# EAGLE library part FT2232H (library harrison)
FT2232H USB to FIFO
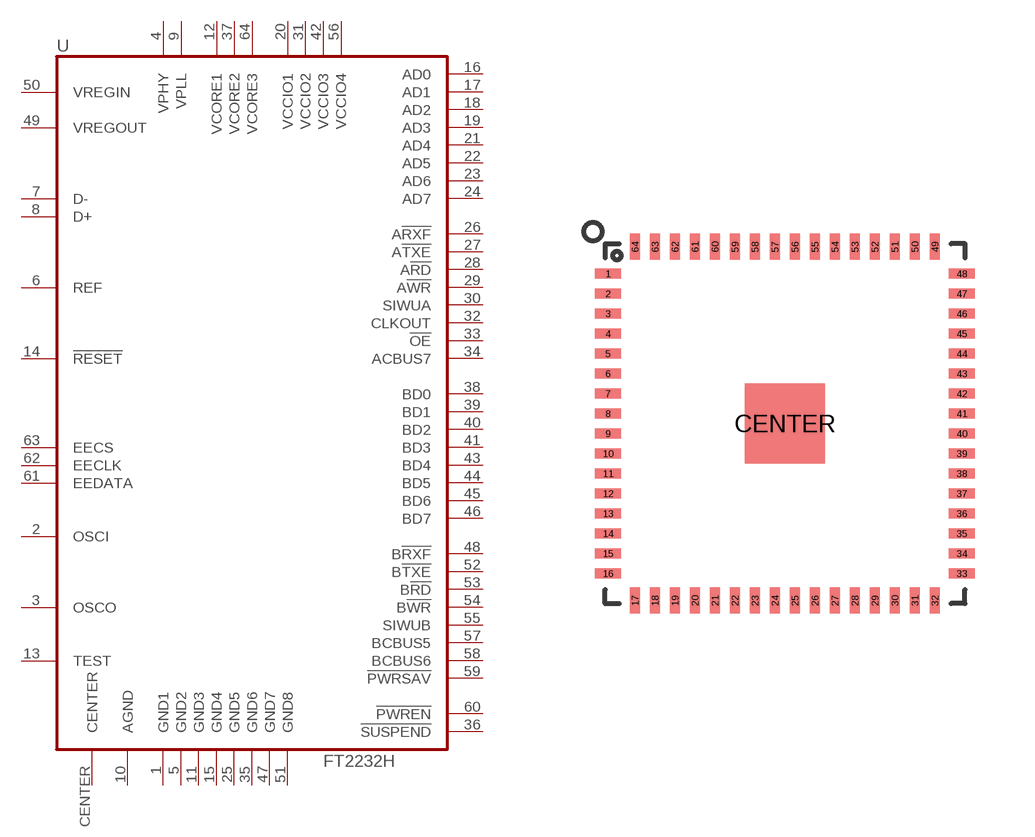
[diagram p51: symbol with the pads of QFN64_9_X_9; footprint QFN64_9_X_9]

Designator prefix U

## FT2232H  [QFN64_9_X_9]
1  GND1  pwr
2  OSCI  in
3  OSCO  out
4  VPHY  pwr
5  GND2  pwr
6  REF  pas
7  D-
8  D+
9  VPLL  pwr
10  AGND  pwr
11  GND3  pwr
12  VCORE1  pwr
13  TEST  in
14  !RESET!  in
15  GND4  pwr
16  AD0
17  AD1
18  AD2
19  AD3
20  VCCIO1  pwr
21  AD4
22  AD5
23  AD6
24  AD7
25  GND5  pwr
26  A!RXF!  out
27  A!TXE!  out
28  A!RD!  in
29  A!WR!  in
30  SIWUA  in
31  VCCIO2  pwr
32  CLKOUT  out
33  !OE!  in
34  ACBUS7
35  GND6  pwr
36  !SUSPEND!  out
37  VCORE2  pwr
38  BD0
39  BD1
40  BD2
41  BD3
42  VCCIO3  pwr
43  BD4
44  BD5
45  BD6
46  BD7
47  GND7  pwr
48  B!RXF!  out
49  VREGOUT  pwr
50  VREGIN  pwr
51  GND8  pwr
52  B!TXE!  out
53  B!RD!  in
54  B!WR!  in
55  SIWUB  in
56  VCCIO4  pwr
57  BCBUS5
58  BCBUS6
59  !PWRSAV!  in
60  !PWREN!  out
61  EEDATA
62  EECLK  out
63  EECS
64  VCORE3  pwr
CENTER  CENTER  pwr

## Footprint QFN64_9_X_9 (pad centres in mm)
smd 0.65 x 0.25: 1 -4.425,3.75; 2 -4.425,3.25; 3 -4.425,2.75; 4 -4.425,2.25; 5 -4.425,1.75; 6 -4.425,1.25; 7 -4.425,0.75; 8 -4.425,0.25; 9 -4.425,-0.25; 10 -4.425,-0.75; 11 -4.425,-1.25; 12 -4.425,-1.75; 13 -4.425,-2.25; 14 -4.425,-2.75; 15 -4.425,-3.25; 16 -4.425,-3.75; 33 4.425,-3.75; 34 4.425,-3.25; 35 4.425,-2.75; 36 4.425,-2.25; 37 4.425,-1.75; 38 4.425,-1.25; 39 4.425,-0.75; 40 4.425,-0.25; 41 4.425,0.25; 42 4.425,0.75; 43 4.425,1.25; 44 4.425,1.75; 45 4.425,2.25; 46 4.425,2.75; 47 4.425,3.25; 48 4.425,3.75
smd 0.25 x 0.65: 17 -3.75,-4.425; 18 -3.25,-4.425; 19 -2.75,-4.425; 20 -2.25,-4.425; 21 -1.75,-4.425; 22 -1.25,-4.425; 23 -0.75,-4.425; 24 -0.25,-4.425; 25 0.25,-4.425; 26 0.75,-4.425; 27 1.25,-4.425; 28 1.75,-4.425; 29 2.25,-4.425; 30 2.75,-4.425; 31 3.25,-4.425; 32 3.75,-4.425; 49 3.75,4.425; 50 3.25,4.425; 51 2.75,4.425; 52 2.25,4.425; 53 1.75,4.425; 54 1.25,4.425; 55 0.75,4.425; 56 0.25,4.425; 57 -0.25,4.425; 58 -0.75,4.425; 59 -1.25,4.425; 60 -1.75,4.425; 61 -2.25,4.425; 62 -2.75,4.425; 63 -3.25,4.425; 64 -3.75,4.425
smd 2 x 2: CENTER 0,0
